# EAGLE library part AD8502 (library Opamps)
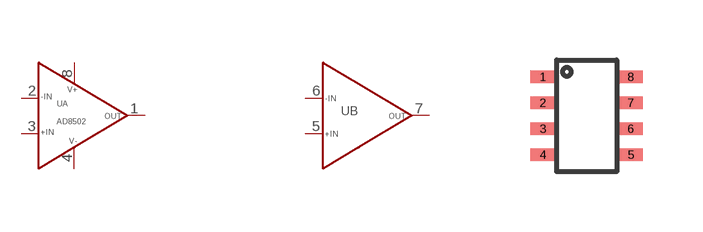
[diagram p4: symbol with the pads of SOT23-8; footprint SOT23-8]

Designator prefix U; gates A=CH1 B=CHGEN

## AD8502  [SOT23-8]
1  A:OUTA
2  A:-INA
3  A:+INA
4  A:GND
5  B:+INB
6  B:-INB
7  B:OUTB
8  A:VCC

## Footprint SOT23-8 (pad centres in mm)
smd 0.61 x 0.305: 1 -1.1,0.975; 2 -1.1,0.325; 3 -1.1,-0.325; 4 -1.1,-0.975; 5 1.1,-0.975; 6 1.1,-0.325; 7 1.1,0.325; 8 1.1,0.975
